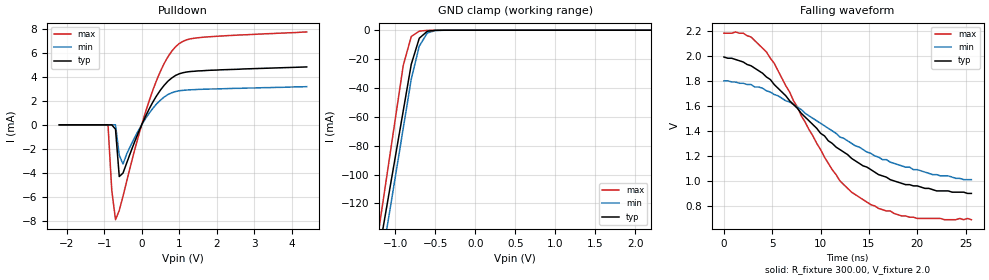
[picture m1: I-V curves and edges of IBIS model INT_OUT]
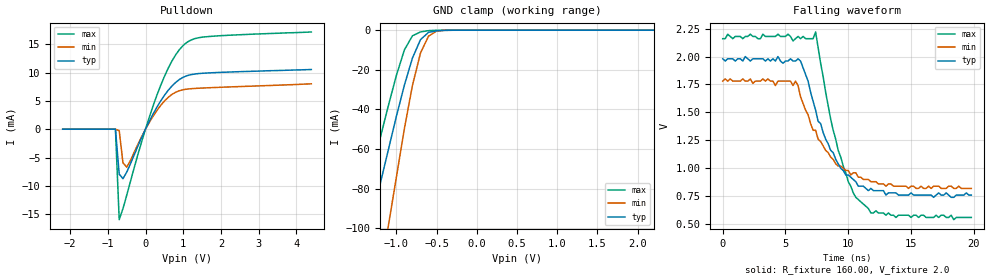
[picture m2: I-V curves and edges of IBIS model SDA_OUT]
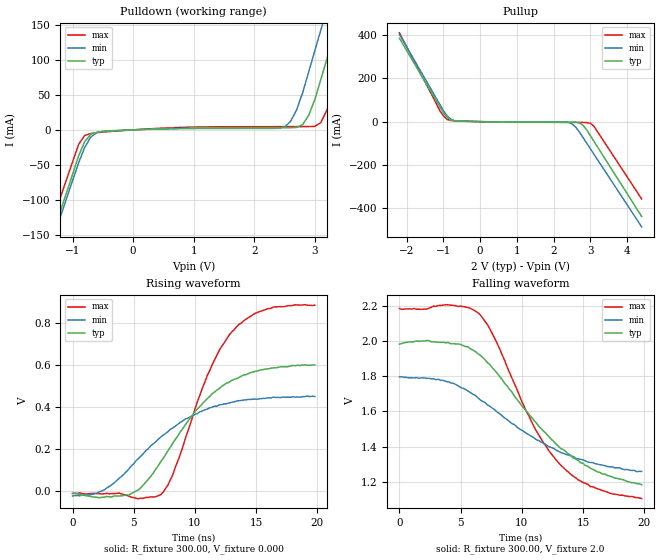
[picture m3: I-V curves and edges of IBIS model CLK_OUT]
| IBIS file 8564nb2v.ibs
[IBIS ver]   3.2
[File name]   8564nb2v.ibs
[File Rev]   1.0
[Date]   Jan 22, 2008
[Source]   This file orginated at EPSON TOYOCOM Corp.
[Copyright]   Copyright EPSON TOYOCOM Corp. 2008
|   Component 8564nb2v
[Component]   8564nb2v
[Manufacturer]   EPSON TOYOCOM
[Package]
| variable   typ   min   max
R_pkg   87m   NA   NA
L_pkg   10nH   NA   NA
C_pkg   206fF   NA   NA
[Pin]  signal_name   model_name   R_pin   L_pin   C_pin
1   /INT   INT_OUT
2   GND   GND
|3   GND
|4   NC
5   SDA   SDA_OUT
6   SCL   SCL_IN
7   CLKOUT   CLK_OUT
8   VDD   POWER
9   CLKOE   OE_IN
|10   NC
|11   NC
|12   NC
|13   NC
|14   NC
|15   NC
|16   NC
|17   NC
|18   NC
|19   NC
|20   NC
|21   NC
|22   NC
5T   SDA   SDA_IN
| Models and submodels in the file (6): INT_OUT (Open_drain), SDA_OUT (Open_drain), CLK_OUT (Output), SCL_IN (Input), OE_IN (Input), SDA_IN (Input)
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|   Model OUTPUT
[Model]   INT_OUT
Model_type   Open_drain
Polarity   Non-Inverting
C_comp   5pF   5pF   5pF
[Temperature Range]   25.00   85.00   -40.000
[Voltage Range]   2.0V   1.8V   2.2V
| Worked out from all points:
|   slope of the pulldown table from 0 to 0.3 V, typ, clamps not added: 158 ohm
|   GND clamp passes 1 mA (typ) near -0.61 V on its own axis
|   falling waveform, R_fixture 300.00, V_fixture 2.0: 20-80 % time 9.3ns typ, 10.5ns min, 6.57ns max; typ from 1.99 V to 0.9 V
[Pulldown]
| voltage   I(typ)   I(min)   I(max)
-2.2V     0A         0A         0A
-900mV    0A         0A         0A
-800mV    0A         0A         -5.44mA
-700mV    -360uA     0A         -7.89mA
-600mV    -4.3mA     -2.53mA    -7.12mA
-500mV    -4.01mA    -3.26mA    -5.94mA
-200mV    -1.49mA    -1.12mA    -2.21mA
200mV     1.34mA     980uA      2.02mA
600mV     3.3mA      2.32mA     5.12mA
900mV     4.11mA     2.77mA     6.49mA
1.5V      4.49mA     2.95mA     7.25mA
4.4V      4.82mA     3.18mA     7.73mA
[GND_clamp]
| voltage   I(typ)   I(min)   I(max)
-2.2V     -474.3mA   -510.3mA   -509.5mA
-1.2V     -152.4mA   -170mA     -136.3mA
-1.1V     -120.2mA   -135.9mA   -99.03mA
-1V       -88.01mA   -101.9mA   -61.71mA
-900mV    -55.82mA   -67.88mA   -24.39mA
-800mV    -23.63mA   -33.85mA   -4.35mA
-700mV    -5.57mA    -11.01mA   -620uA
-600mV    -710uA     -1.96mA    -110uA
-500mV    -80uA      -200uA     -10uA
2.2V      0A         0A         0A
[Ramp]
| variable   typ   min   max
dV/dt_r 0.74/8.0n   0.56/8.0n   0.95/8.0n
dV/dt_f 0.65/9.2n   0.47/10.4n   0.90/10.8n
R_load = 300.00
[Falling Waveform]
R_fixture = 300.00
V_fixture = 2.0
V_fixture_min = 1.8
V_fixture_max = 2.2
| time   V(typ)   V(min)   V(max)
0s        1.99V      1.8V       2.18V
2ns       1.95V      1.78V      2.18V
4.4ns     1.83V      1.72V      2.03V
5.2ns     1.77V      1.69V      1.94V
10.4ns    1.36V      1.44V      1.19V
12ns      1.25V      1.35V      1V
13.2ns    1.18V      1.3V       910mV
16ns      1.05V      1.19V      780mV
18.4ns    980mV      1.12V      720mV
25.6ns    900mV      1.01V      690mV
[Model]   SDA_OUT
Model_type   Open_drain
Polarity   Non-Inverting
C_comp   5pF   5pF   5pF
[Temperature Range]   25.00   85.00   -40.000
[Voltage Range]   2.0V   1.8V   2.2V
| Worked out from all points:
|   slope of the pulldown table from 0 to 0.3 V, typ, clamps not added: 78.1 ohm
|   GND clamp passes 1 mA (typ) near -0.59 V on its own axis
|   falling waveform, R_fixture 160.00, V_fixture 2.0: 20-80 % time 2.49ns typ, 3.11ns min, 2.03ns max; typ from 1.98 V to 0.76 V
[Pulldown]
| voltage   I(typ)   I(min)   I(max)
-2.2V     0A         0A         0A
-800mV    0A         0A         0A
-700mV    -7.92mA    -250uA     -15.95mA
-600mV    -8.72mA    -5.93mA    -13.99mA
-500mV    -7.56mA    -6.69mA    -11.62mA
-100mV    -1.4mA     -1.25mA    -2.11mA
300mV     3.88mA     3.3mA      5.99mA
700mV     7.62mA     6.14mA     12.03mA
1V        9.17mA     6.97mA     14.78mA
1.2V      9.62mA     7.14mA     15.71mA
1.6V      9.9mA      7.29mA     16.3mA
4.4V      10.53mA    8.01mA     17.15mA
[GND_clamp]
| voltage   I(typ)   I(min)   I(max)
-2.2V     -246.7mA   -369.2mA   -215.6mA
-1.5V     -128.1mA   -197.1mA   -102.7mA
-1.4V     -111.2mA   -172.6mA   -86.53mA
-1.3V     -94.28mA   -148mA     -70.4mA
-1.1V     -60.42mA   -98.82mA   -38.14mA
-1V       -43.49mA   -74.24mA   -22.85mA
-900mV    -27.68mA   -49.66mA   -9.91mA
-800mV    -14.03mA   -27.81mA   -2.79mA
-700mV    -4.76mA    -11.5mA    -870uA
-600mV    -1.07mA    -2.98mA    -200uA
-500mV    -320uA     -440uA     -10uA
2.2V      0A         0A         0A
[Ramp]
| variable   typ   min   max
dV/dt_r 0.77/2.2n   0.61/2.2n   0.91/2.0n
dV/dt_f 0.76/2.8n   0.59/3.0n   1.01/2.2n
R_load = 160.00
[Falling Waveform]
R_fixture = 160.00
V_fixture = 2.0
V_fixture_min = 1.8
V_fixture_max = 2.2
| time   V(typ)   V(min)   V(max)
0s        1.98V      1.78V      2.16V
6ns       1.98V      1.74V      2.18V
6.8ns     1.78V      1.48V      2.16V
7.4ns     1.52V      1.34V      2.22V
8.8ns     1.14V      1.08V      1.34V
10ns      940mV      980mV      880mV
10.6ns    880mV      960mV      740mV
11.8ns    820mV      880mV      600mV
13.8ns    780mV      840mV      560mV
19.8ns    760mV      820mV      560mV
[Model]   CLK_OUT
Model_type   Output
Polarity   Non-Inverting
Enable   Active-High
Vmeas =   1.50V
C_comp   1.69pF   1.32pF   1.96pF
[Temperature Range]   25.00   85.00   -40.000
[Voltage Range]   2.0V   1.8V   2.2V
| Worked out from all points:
|   slope of the pulldown table from 0 to 0.3 V, typ, clamps not added: 268 ohm
|   slope of the pullup table from 0 to 0.3 V, typ, clamps not added: 316 ohm
|   rising waveform, R_fixture 300.00, V_fixture 0.000: 20-80 % time 4.86ns typ, 5.66ns min, 3.63ns max; typ from -0.009 V to 0.6 V
|   falling waveform, R_fixture 300.00, V_fixture 2.0: 20-80 % time 6.19ns typ, 6.96ns min, 4.76ns max; typ from 1.98 V to 1.18 V
[Pulldown]
| voltage   I(typ)   I(min)   I(max)
-2.2V     -378.9mA   -379mA     -347mA
-1.4V     -168.6mA   -174.7mA   -146.2mA
-1.3V     -142.3mA   -149.1mA   -121.1mA
-900mV    -37.1mA    -46.97mA   -20.7mA
-700mV    -6.4mA     -10.43mA   -5.19mA
2.5V      3.04mA     3.89mA     4.58mA
2.8V      7.52mA     52.87mA    4.63mA
3V        42.83mA    112.5mA    4.94mA
3.1V      71.88mA    142.3mA    10.31mA
3.3V      130mA      201.9mA    54.39mA
3.6V      217.1mA    291.3mA    153.1mA
4.4V      449.5mA    529.8mA    416.3mA
[Pullup]
| voltage   I(typ)   I(min)   I(max)
-2.2V     385.9mA    403.8mA    411.1mA
-1.1V     69.28mA    80.2mA     50.53mA
-900mV    19.33mA    26.64mA    10.09mA
-800mV    7.03mA     11.36mA    5.17mA
-600mV    2.77mA     2.34mA     3.61mA
2.3V      -2.34mA    -1.99mA    -3.32mA
2.5V      -2.5mA     -10.02mA   -3.37mA
2.7V      -5.79mA    -47.19mA   -3.46mA
2.8V      -16.59mA   -73.06mA   -3.69mA
3V        -64.15mA   -124.8mA   -7.37mA
3.1V      -90.92mA   -150.7mA   -21.33mA
4.4V      -438.9mA   -487mA     -357.8mA
[Ramp]
| variable   typ   min   max
dV/dt_r 0.343/5.4n   0.258/6.2n   0.502/4.2n
dV/dt_f 0.428/6.2n   0.324/6.8n   0.663/4.4n
R_load = 300.00
[Rising Waveform]
R_fixture = 300.00
V_fixture = 0.000
| time   V(typ)   V(min)   V(max)
0s        -8.94mV    -21.52mV   -9.11mV
2.6ns     -27.09mV   8.11mV     -10.86mV
4.6ns     -16.53mV   106.1mV    -21.9mV
5.6ns     18.63mV    168.6mV    -31.87mV
7.2ns     139.8mV    257.2mV    -15.37mV
8.2ns     229.6mV    301.5mV    79.34mV
11ns      439.2mV    390.2mV    548mV
13ns      526.3mV    422.1mV    755.6mV
16ns      581.5mV    443.9mV    867mV
19.8ns    599.7mV    450.1mV    882.8mV
[Falling Waveform]
R_fixture = 300.00
V_fixture = 2.0
V_fixture_min = 1.8
V_fixture_max = 2.2
| time   V(typ)   V(min)   V(max)
0s        1.984V     1.797V     2.186V
2.2ns     2.004V     1.789V     2.183V
3.6ns     1.994V     1.777V     2.206V
5ns       1.982V     1.736V     2.2V
6.4ns     1.93V      1.679V     2.163V
7.8ns     1.834V     1.61V      2.015V
11ns      1.549V     1.45V      1.514V
13ns      1.402V     1.373V     1.308V
15.6ns    1.277V     1.309V     1.172V
19.8ns    1.183V     1.259V     1.103V
